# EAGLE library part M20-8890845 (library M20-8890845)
2.54mm (0.1") Pitch SIL SMT Horizontal Pin Header, 2.5mm housing height, gold, 8 contacts Source: Datasheet
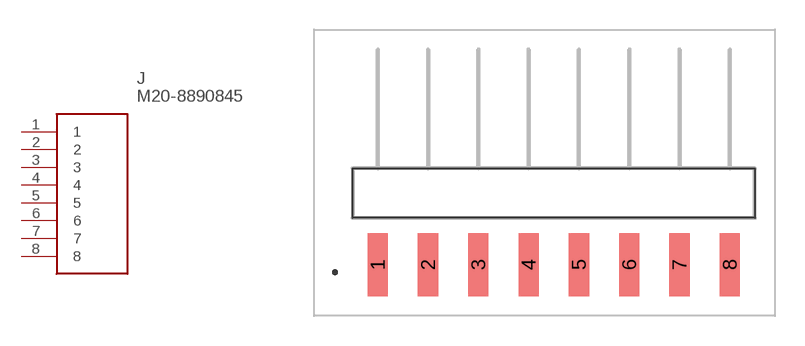
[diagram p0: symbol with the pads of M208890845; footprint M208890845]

Designator prefix J

## M20-8890845 (Description: 2.54mm (0.1") Pitch SIL SMT Horizontal Pin Header, 2.5mm housing height, gold, 8 contacts; Height: mm; Manufacturer_Name: Harwin; Manufacturer_Part_Number: M20-8890845; Mouser_Part_Number: 855-M20-8890845; Mouser_Price-Stock: https://www.mouser.co.uk/ProductDetail/Harwin/M20-8890845?qs=k41KVqW3ymqbj55BP%2FIx8Q%3D%3D)  [M208890845]
1  1
2  2
3  3
4  4
5  5
6  6
7  7
8  8

## Footprint M208890845 (pad centres in mm)
M20-8890845-1
smd 1.02 x 3.17: 1 -8.89,-3.615; 2 -6.35,-3.615; 3 -3.81,-3.615; 4 -1.27,-3.615; 5 1.27,-3.615; 6 3.81,-3.615; 7 6.35,-3.615; 8 8.89,-3.615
